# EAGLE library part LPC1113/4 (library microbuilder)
LPC1113/4 MCU QFP48 Package ARM Cortex M0, 50MHz Operation, 8 Channel 10-Bit ADC, 1²C, 2xSPI, UART, 2x16 Bit and 2x32 Bit Timers, Internal 12MHz Oscillator, 1.8-3.6V operation. Model Flash SRAM Part N°: Digikey Mouser LPC1113 24KB 8KB LPC1113FBD48/301 TBD TBD LPC1114 32KB 8KB LPC1114FBD48/301 568-4950-ND 771-LPC1114FBD483011
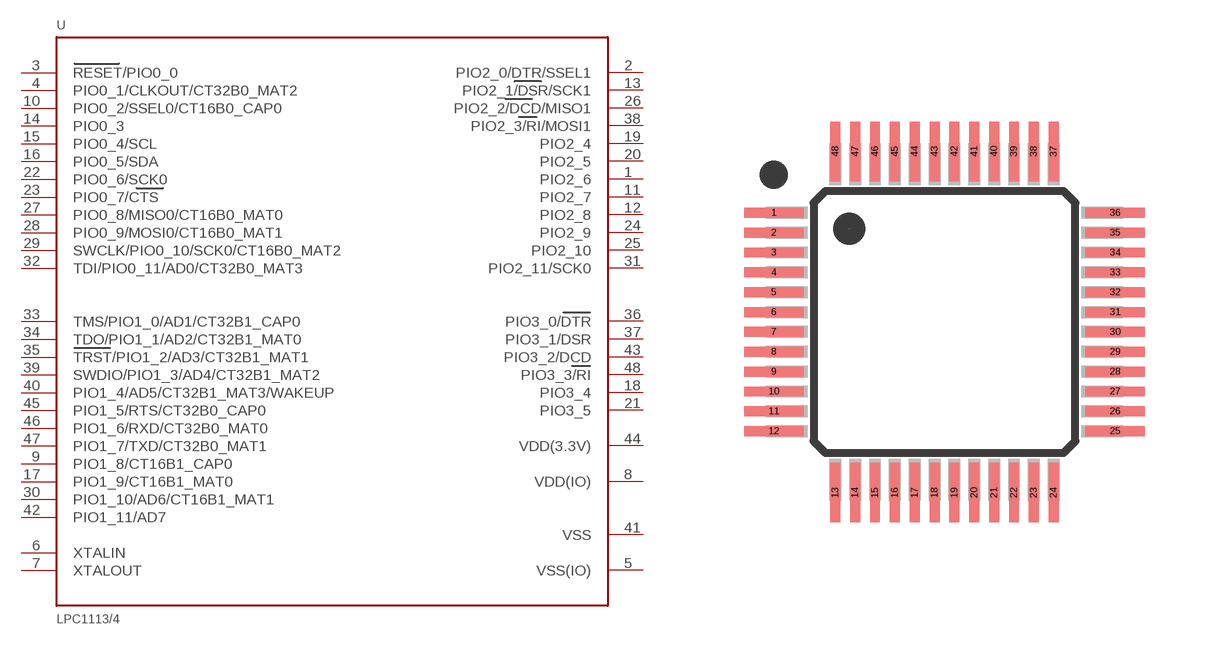
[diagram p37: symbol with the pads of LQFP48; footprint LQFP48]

Designator prefix U

## LPC1113/4 (DIGIKEY#: 568-4950-ND; MANF: NXP; MANF#: LPC1114FBD48/301,1)  [LQFP48]
1  PIO2_6
2  PIO2_0/DTR/SSEL1
3  RESET/PIO0_0
4  PIO0_1/CLKOUT/CT32B0_MAT2
5  VSS(IO)  pwr
6  XTALIN  in
7  XTALOUT  out
8  VDD(IO)  pwr
9  PIO1_8/CT16B1_CAP0
10  PIO0_2/SSEL0/CT16B0_CAP0
11  PIO2_7
12  PIO2_8
13  PIO2_1/DSR/SCK1
14  PIO0_3
15  PIO0_4/SCL
16  PIO0_5/SDA
17  PIO1_9/CT16B1_MAT0
18  PIO3_4
19  PIO2_4
20  PIO2_5
21  PIO3_5
22  PIO0_6/SCK0
23  PIO0_7/CTS
24  PIO2_9
25  PIO2_10
26  PIO2_2/DCD/MISO1
27  PIO0_8/MISO0/CT16B0_MAT0
28  PIO0_9/MOSI0/CT16B0_MAT1
29  SWCLK/PIO0_10/SCK0/CT16B0_MAT2
30  PIO1_10/AD6/CT16B1_MAT1
31  PIO2_11/SCK0
32  TDI/PIO0_11/AD0/CT32B0_MAT3
33  TMS/PIO1_0/AD1/CT32B1_CAP0
34  TDO/PIO1_1/AD2/CT32B1_MAT0
35  TRST/PIO1_2/AD3/CT32B1_MAT1
36  PIO3_0/DTR
37  PIO3_1/DSR
38  PIO2_3/RI/MOSI1
39  SWDIO/PIO1_3/AD4/CT32B1_MAT2
40  PIO1_4/AD5/CT32B1_MAT3/WAKEUP
41  VSS  pwr
42  PIO1_11/AD7
43  PIO3_2/DCD
44  VDD(3.3V)  pwr
45  PIO1_5/RTS/CT32B0_CAP0
46  PIO1_6/RXD/CT32B0_MAT0
47  PIO1_7/TXD/CT32B0_MAT1
48  PIO3_3/RI

## Footprint LQFP48 (pad centres in mm)
smd 1.5 x 0.25: 1 -4.3,2.75; 2 -4.3,2.25; 3 -4.3,1.75; 4 -4.3,1.25; 5 -4.3,0.75; 6 -4.3,0.25; 7 -4.3,-0.25; 8 -4.3,-0.75; 9 -4.3,-1.25; 10 -4.3,-1.75; 11 -4.3,-2.25; 12 -4.3,-2.75; 25 4.3,-2.75; 26 4.3,-2.25; 27 4.3,-1.75; 28 4.3,-1.25; 29 4.3,-0.75; 30 4.3,-0.25; 31 4.3,0.25; 32 4.3,0.75; 33 4.3,1.25; 34 4.3,1.75; 35 4.3,2.25; 36 4.3,2.75
smd 0.25 x 1.5: 13 -2.75,-4.3; 14 -2.25,-4.3; 15 -1.75,-4.3; 16 -1.25,-4.3; 17 -0.75,-4.3; 18 -0.25,-4.3; 19 0.25,-4.3; 20 0.75,-4.3; 21 1.25,-4.3; 22 1.75,-4.3; 23 2.25,-4.3; 24 2.75,-4.3; 37 2.75,4.3; 38 2.25,4.3; 39 1.75,4.3; 40 1.25,4.3; 41 0.75,4.3; 42 0.25,4.3; 43 -0.25,4.3; 44 -0.75,4.3; 45 -1.25,4.3; 46 -1.75,4.3; 47 -2.25,4.3; 48 -2.75,4.3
